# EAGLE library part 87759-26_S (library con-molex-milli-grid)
HEADER
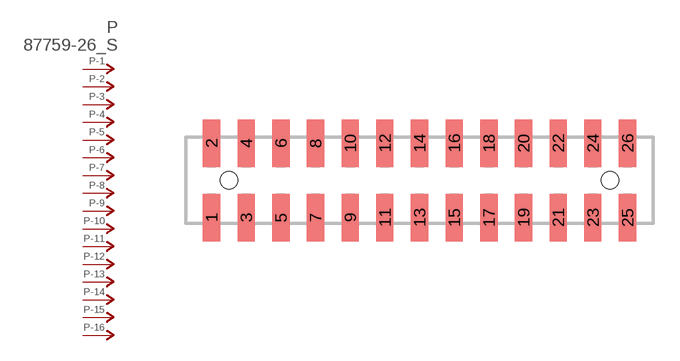
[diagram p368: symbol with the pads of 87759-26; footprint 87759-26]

Designator prefix P; gates -1=P-NV -2=P-N -3=P-N -4=P-N -5=P-N -6=P-N -7=P-N -8=P-N -9=P-N -10=P-N -11=P-N -12=P-N -13=P-N -14=P-N -15=P-N -16=P-N -17=P-N -18=P-N -19=P-N -20=P-N -21=P-N -22=P-N -23=P-N -24=P-N -25=P-N -26=P-N

## 87759-26_S  [87759-26]
1  -1:P  pas
2  -2:P  pas
3  -3:P  pas
4  -4:P  pas
5  -5:P  pas
6  -6:P  pas
7  -7:P  pas
8  -8:P  pas
9  -9:P  pas
10  -10:P  pas
11  -11:P  pas
12  -12:P  pas
13  -13:P  pas
14  -14:P  pas
15  -15:P  pas
16  -16:P  pas
17  -17:P  pas
18  -18:P  pas
19  -19:P  pas
20  -20:P  pas
21  -21:P  pas
22  -22:P  pas
23  -23:P  pas
24  -24:P  pas
25  -25:P  pas
26  -26:P  pas

## Footprint 87759-26 (pad centres in mm)
HEADER SMD Dual Row, Vertical
smd 1 x 2.75: 1 -12,-2.15; 2 -12,2.15; 3 -10,-2.15; 4 -10,2.15; 5 -8,-2.15; 6 -8,2.15; 7 -6,-2.15; 8 -6,2.15; 9 -4,-2.15; 10 -4,2.15; 11 -2,-2.15; 12 -2,2.15; 13 0,-2.15; 14 0,2.15; 15 2,-2.15; 16 2,2.15; 17 4,-2.15; 18 4,2.15; 19 6,-2.15; 20 6,2.15; 21 8,-2.15; 22 8,2.15; 23 10,-2.15; 24 10,2.15; 25 12,-2.15; 26 12,2.15
hole 1 at -11,0
hole 1 at 11,0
